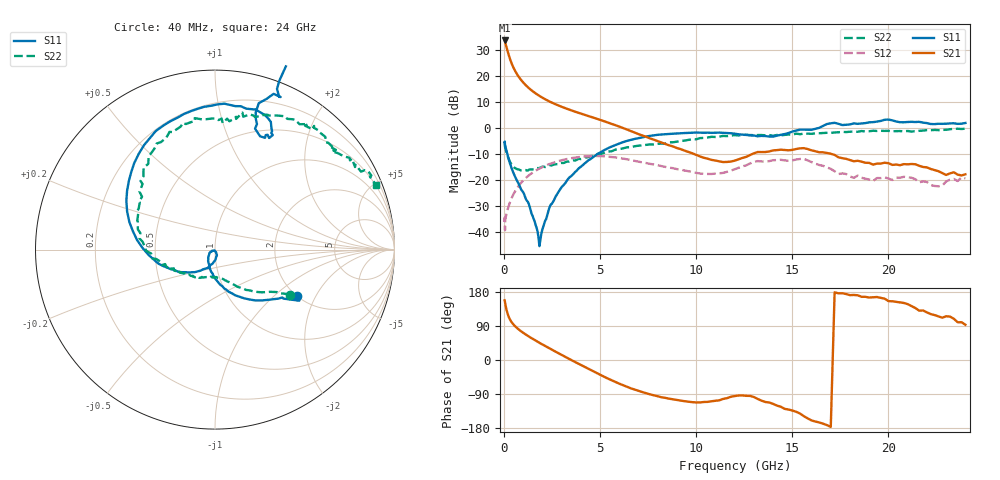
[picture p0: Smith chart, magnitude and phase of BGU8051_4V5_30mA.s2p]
! BGU8051_4V5_30mA
! Date/time Tue Jun 16 10:58:09 2015
! VAR V_out= 4.5000
! VAR I_out= 29.9450
! VAR V_in= 3.7520
! VAR I_in= 0.3927
# MHz S MA R 50
!  Freq-MHz  S11-mag  S11-arg  S21-mag  S21-arg  S12-mag  S12-arg  S22-mag  S22-arg
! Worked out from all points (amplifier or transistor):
!   187 points, 40 MHz to 24 GHz, reference 50 ohm
!   highest |S21| = 33.6 dB at 40 MHz (marker M1)
!   |S21| within 3 dB of that: start of sweep to 155.4 MHz
!   unconditionally stable (mu >= 1): 635.7 MHz to 14.07 GHz
!   at 750 MHz: K = 1.01, MAG = 20.6 dB, |S12| = -22.4 dB
!   at 5.4 GHz: K = 1.21, MAG = 3.8 dB, |S12| = -11.0 dB
!   at 24 GHz: K = -0.59, MSG = 0.8 dB, |S12| = -19.3 dB
!   lowest NFmin = 0.30 dB at 400 MHz
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40  0.5254 -29.5  47.68 157.5  0.0158 33.9  0.4868 -31.4
50  0.549 -31.2  46.32 155.6  0.01916 -13.1  0.4692 -31.7
60  0.469 -35.6  45.52 152.4  0.01089 24.6  0.4355 -33.9
80  0.4472 -37.6  42.49 147.0  0.01774 36.0  0.4028 -35.8
120  0.3877 -46.9  37.76 136.8  0.02107 40.5  0.354 -42.2
180  0.3144 -59.4  31.23 124.8  0.02554 48.4  0.2978 -49.7
240  0.2599 -69.1  26.09 115.6  0.03059 52.5  0.2585 -55.8
300  0.2218 -76.7  22.16 108.7  0.03597 54.7  0.2303 -60.2
360  0.1872 -83.6  19.12 103.2  0.04074 56.5  0.2088 -64.1
440  0.1542 -91.2  16.09 97.4  0.04784 58.1  0.1907 -68.9
550  0.1236 -100.3  13.2 90.8  0.05768 58.7  0.1724 -73.7
750  0.08731 -112.8  9.88 81.6  0.07547 57.5  0.1601 -81.8
950  0.0622 -127.3  7.885 73.8  0.09304 55.1  0.153 -88.5
1600  0.01614 -155.8  4.75 52.7  0.1471 43.6  0.1625 -108.9
1850  0.005381 -116.6  4.116 45.4  0.1662 38.6  0.1707 -116.0
2600  0.0407 -80.6  2.94 24.4  0.2171 22.7  0.1985 -132.1
4100  0.192 -138.3  1.835 -15.7  0.2811 -10.4  0.2558 -155.4
8200  0.749 112.5  0.5242 -98.4  0.1853 -76.8  0.5001 147.9
12200  0.7558 65.5  0.2494 -93.7  0.1719 -71.7  0.7182 103.1
16200  0.9598 68.9  0.3572 -162.4  0.2062 -150.6  0.7888 71.0
20200  1.397 34.2  0.1951 154.9  0.1003 -158.8  0.859 44.1
24000  1.243 20.9  0.1288 93.1  0.1081 -173.3  0.9677 21.7
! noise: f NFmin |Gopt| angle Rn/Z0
400  0.2955  0.1705  21.92  0.052
550  0.3099  0.1418  32.35  0.052
950  0.3585  0.1004  72.67  0.0511
1250  0.4047  0.1032  105  0.0501
1600  0.4692  0.1243  131.2  0.049
1900  0.5335  0.1452  146.4  0.0484
2250  0.6191  0.1678  160.2  0.0487
2600  0.7161  0.1885  172  0.0504
3300  0.9443  0.2299  192.5  0.0601
4000  1.218  0.2793  209.2  0.0815
